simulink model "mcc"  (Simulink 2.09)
settings: Solver=ode45  StartTime=0.0  StopTime=10.0  RelTol=1e-3  AbsTol=1e-6

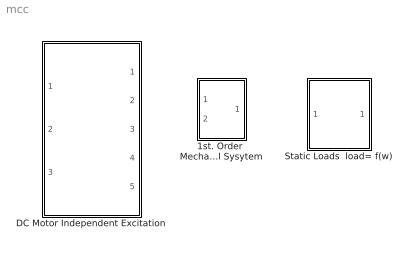
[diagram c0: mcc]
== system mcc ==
  1st. Order  Mechanical Sysytem : Subsystem  mask(First Order Mechanical System){J=15, b=.005, wor=0}
      mask prompts: J "Inertia [Kgm]:"; b "Friction Coeficient [Nm seg/rad]:"; wor "Speed Initial Condition [rad/sec]:"
      mask help: This block solves the following differential equation: dW(t)/dt = - W(t)/J + (Tm - Load )/J W(0)=W0
  DC Motor Independent Excitation : Subsystem  mask(DC Motor ){La=3e-3, Ra=.05, Re=25.2, Ie=[ 0 4.3 5.3 6.2 7.3 8 8.8 10.5], phy=[0 286.5 334.25 382 424 453.62 477.5 525.25], k=.016, ciia=0, f0=0}
      mask prompts: La "Armature Inductance  [Hy]:"; Ra "Armature Resistance [Ohms]:"; Re "Field Resistance  [Ohms]:"; Ie "Field Current Vector [Amp]:"; phy "Field Flux Vector [Wb]:"; k "Motor Constant:"; ciia "Armature Current Initial Condition [Amp]:"; f0 "Flux Initial Condition [Wb]"
  Static Loads  load= f(w) : Subsystem  mask(Load Torques){w=1, Tn=1, c=Centrifugal Pumps}
      mask prompts: w "Rated Speed [rad/sec]:"; Tn "Rated Torque [N*m]:"; c "Load Type:"
      mask help: This block generates at its output a Load torque which is a function of the rotational speed. The block icon displays the load characteristic in use. The left edge of the icon represents the load from 0 to 100% of ratred load, and the lower edge represents the speed from 0 to 100% rated speed.
      mask init:
      | switch c
      | case 1
      | x=[0  1];
      | y=[1 1];
      | case 2
      | x=[0 1 1.5 2 3 4 5 6 10];
      | y=[1.22 .98 .91 .92 .95 .97 .98 1 1];
      | case 3
      | x=[0 1 2 3 4 5 6 7 8 9 10];
      | y=[1 .87 .84 .85 .88 .9 .92 .94 .96 .98 1];
      | case 4
      | x=[0 1 2 3 4 5 6 7 8 9 10];
      | y=[1.3 1.1 .98 .95 .94 .945 .95 .96 .97 .98 1];
      | case 5
      | x=[0 1 2 3 4 5 6 7 8 9 10];
      | y=[1.3 1.1 .98 .95 .94 .945 .95 .96 .97 .98 1];
      | case 6
      | x=[0 1 2 3 4 5 6 7 8 9 10];
      | y=[.5 .36 .34 .36 .44 .5 .6 .7 .8 .9 1];
      | case 7
      | x=[0 .5 .50001 1 2 3 4 5 6 7 8 9 10];
      | y=[0 0 .08 .05 .04 .1 .17 .24 .36 .47 .62 .8 1];
      | case 8
      | x=[0 .5 .50001 1 2 3 4 5 6 7 8 9 10];
      | y=[0 0 .08 .05 .04 .1 .17 .24 .36 .47 .62 .8 1];
      | end

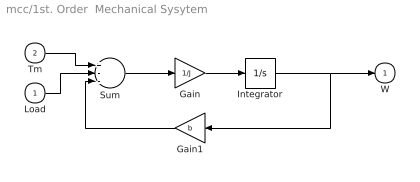
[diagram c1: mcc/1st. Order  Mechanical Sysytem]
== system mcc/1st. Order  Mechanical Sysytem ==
  Load : Inport  Port=1  PortWidth=-1  SampleTime=-1
  Tm : Inport  Port=2  PortWidth=-1  SampleTime=-1
  Gain : Gain  Gain=1/J
  Gain1 : Gain  Orientation=left  Gain=b
  Integrator : Integrator  ExternalReset=none  InitialConditionSource=internal  InitialCondition=wor  LimitOutput=off  UpperSaturationLimit=inf  LowerSaturationLimit=-inf  ShowSaturationPort=off  ShowStatePort=off  AbsoluteTolerance=auto
  Sum : Sum  Inputs=+--
  W : Outport  Port=1  InitialOutput=0
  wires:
  Load/1 -> Sum/2
  Tm/1 -> Sum/1
  Sum/1 -> Gain/1
  Gain/1 -> Integrator/1
  Gain1/1 -> Sum/3
  Integrator/1 -> Gain1/1, W/1

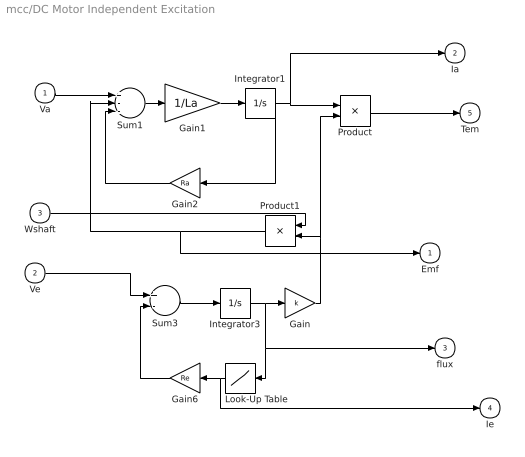
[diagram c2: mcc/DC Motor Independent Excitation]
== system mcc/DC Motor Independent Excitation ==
  Va : Inport  Port=1  PortWidth=-1  SampleTime=-1
  Ve : Inport  Port=2  PortWidth=-1  SampleTime=-1
  Wshaft : Inport  Port=3  PortWidth=-1  SampleTime=-1
  Gain : Gain  Gain=k
  Gain1 : Gain  Gain=1/La
  Gain2 : Gain  Orientation=left  Gain=Ra
  Gain6 : Gain  Orientation=left  Gain=Re
  Integrator1 : Integrator  ExternalReset=none  InitialConditionSource=internal  InitialCondition=ciia  LimitOutput=off  UpperSaturationLimit=inf  LowerSaturationLimit=-inf  ShowSaturationPort=off  ShowStatePort=off  AbsoluteTolerance=auto
  Integrator3 : Integrator  ExternalReset=none  InitialConditionSource=internal  InitialCondition=f0  LimitOutput=off  UpperSaturationLimit=inf  LowerSaturationLimit=-inf  ShowSaturationPort=off  ShowStatePort=off  AbsoluteTolerance=auto
  Look-Up Table : Lookup  Orientation=left  InputValues=phy  OutputValues=Ie
  Product : Product  Inputs=2
  Product1 : Product  Orientation=left  Inputs=2
  Sum1 : Sum  Inputs=+--
  Sum3 : Sum  Inputs=+-
  Emf : Outport  Port=1  InitialOutput=0
  Ia : Outport  Port=2  InitialOutput=0
  flux : Outport  Port=3  InitialOutput=0
  Ie : Outport  Port=4  InitialOutput=0
  Tem : Outport  Port=5  InitialOutput=0
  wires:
  Ve/1 -> Sum3/1
  Wshaft/1 -> Product1/1
  Va/1 -> Sum1/1
  Product/1 -> Tem/1
  Gain/1 -> Product1/2, Product/2
  Integrator3/1 -> flux/1, Look-Up Table/1, Gain/1
  Sum3/1 -> Integrator3/1
  Product1/1 -> Emf/1, Sum1/2
  Integrator1/1 -> Ia/1, Product/1, Gain2/1
  Gain2/1 -> Sum1/3
  Gain1/1 -> Integrator1/1
  Sum1/1 -> Gain1/1
  Gain6/1 -> Sum3/2
  Look-Up Table/1 -> Ie/1, Gain6/1

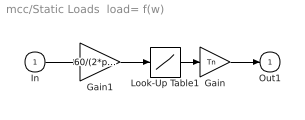
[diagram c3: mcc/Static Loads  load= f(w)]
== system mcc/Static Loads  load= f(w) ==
  In : Inport  Port=1  PortWidth=-1  SampleTime=-1
  Gain : Gain  Gain=Tn
  Gain1 : Gain  Gain=60/(2*pi*w)
  Look-Up Table1 : Lookup  InputValues=x  OutputValues=y
  Out1 : Outport  Port=1  InitialOutput=0
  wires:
  Look-Up Table1/1 -> Gain/1
  Gain/1 -> Out1/1
  In/1 -> Gain1/1
  Gain1/1 -> Look-Up Table1/1
